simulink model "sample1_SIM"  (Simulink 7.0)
settings: Solver=ode3  StartTime=0.0  StopTime=70  RelTol=1e-3
libraries: simulink x6

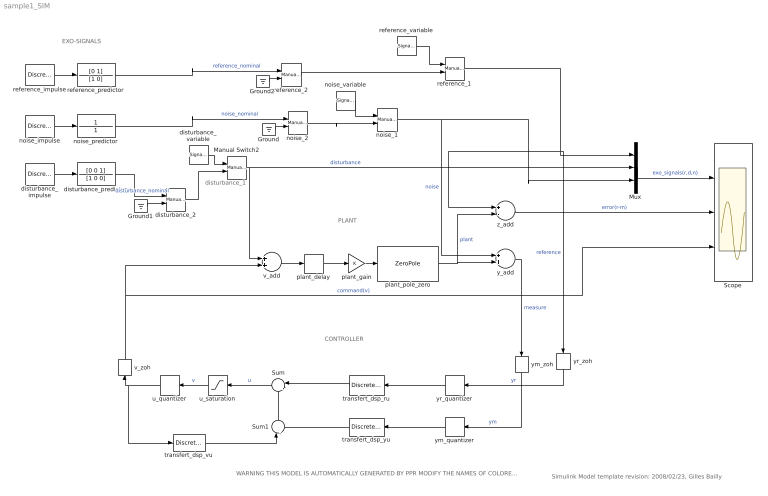
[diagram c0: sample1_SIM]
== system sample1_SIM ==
  note: PLANT
  note: EXO-SIGNALS
  note: Simulink Model template revision: 2008/02/23, Gilles Bailly
  note: CONTROLLER
  note: WARNING THIS MODEL IS AUTOMATICALLY GENERATED BY PPR MODIFY THE NAMES OF COLORED BLOCKS BREAK THIS LINK
  note: disturbance_1
  Ground : Ground
  Ground1 : Ground
  Ground2 : Ground
  Manual Switch2 : simulink/Signal Routing/Manual Switch  SystemSampleTime=-1  sw=0  action=0  varsize=off
  Mux : Mux  Inputs=3
  Scope : Scope  NumInputPorts=3
  Sum : Sum  Orientation=left  Inputs=|+-  OutDataType=sfix(16)  OutScaling=2^0
  Sum1 : Sum  Orientation=up  Inputs=|++  OutDataType=sfix(16)  OutScaling=2^0
  disturbance_2 : simulink/Signal Routing/Manual Switch  SystemSampleTime=-1  sw=1  action=0  varsize=off
  disturbance_impulse : DiscretePulseGenerator  Period=500  PhaseDelay=100  SampleTime=0.1
  disturbance_predictor : TransferFcn  Numerator=[0 0 1]  Denominator=[1 0 0]
  disturbance_variable : SignalGenerator
  noise_1 : simulink/Signal Routing/Manual Switch  SystemSampleTime=-1  sw=0  action=0  varsize=off
  noise_2 : simulink/Signal Routing/Manual Switch  SystemSampleTime=-1  sw=1  action=0  varsize=off
  noise_impulse : DiscretePulseGenerator  Period=500  PhaseDelay=200  SampleTime=0.1
  noise_predictor : TransferFcn  Numerator=1  Denominator=1
  noise_variable : SignalGenerator
  plant_delay : TransportDelay  DelayTime=0.5
  plant_gain : Gain  ParameterDataType=sfix(16)  ParameterScaling=2^0  OutDataType=sfix(16)  OutScaling=2^0
  plant_pole_zero : ZeroPole  Zeros=zeros(0,1)  Poles=-1  Gain=1
  reference_1 : simulink/Signal Routing/Manual Switch  SystemSampleTime=-1  sw=0  action=0  varsize=off
  reference_2 : simulink/Signal Routing/Manual Switch  SystemSampleTime=-1  sw=1  action=0  varsize=off
  reference_impulse : DiscretePulseGenerator  Period=500  PhaseDelay=10  SampleTime=0.1
  reference_predictor : TransferFcn  Numerator=[0 1]  Denominator=[1 0]
  reference_variable : SignalGenerator
  transfert_dsp_ru : DiscreteFilter  Orientation=left  Numerator=[0 0.7104960446]  Denominator=[1 -0.7408182207]  SampleTime=0.1
  transfert_dsp_vu : DiscreteFilter  Numerator=[0 0.1657069833 -0.2998382185 0.1356354391 7.122080703e-014 6.4420691e-014 5.825895322e-014 -0.07062683959 0.06825879814]  Denominator=[1 -2.714285714 2.455782313 -0.740632761 0 0 0 0 0]  SampleTime=0.1
  transfert_dsp_yu : DiscreteFilter  Orientation=left  Numerator=[0 0.7421702746 -1.388829544 0.6490273109]  Denominator=[1 -2.714285714 2.455782313 -0.740632761]  SampleTime=0.1
  u_quantizer : Quantizer  Orientation=left  QuantizationInterval=eps
  u_saturation : Saturate  Orientation=left  UpperLimit=10  LowerLimit=-10
  v_add : Sum  OutDataType=sfix(16)  OutScaling=2^-10
  v_zoh : ZeroOrderHold  Orientation=up  SampleTime=0.1
  y_add : Sum  OutDataType=sfix(16)  OutScaling=2^-10
  ym_quantizer : Quantizer  Orientation=left  QuantizationInterval=eps
  ym_zoh : ZeroOrderHold  Orientation=down  SampleTime=0.1
  yr_quantizer : Quantizer  Orientation=left  QuantizationInterval=eps
  yr_zoh : ZeroOrderHold  Orientation=down  SampleTime=0.1
  z_add : Sum  Inputs=+-  OutDataType=sfix(16)  OutScaling=2^-10
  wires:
  v_add/1 -> plant_delay/1
  y_add/1 -> ym_zoh/1  "measure"
  reference_impulse/1 -> reference_predictor/1
  noise_impulse/1 -> noise_predictor/1
  disturbance_impulse/1 -> disturbance_predictor/1
  plant_delay/1 -> plant_gain/1
  plant_gain/1 -> plant_pole_zero/1
  plant_pole_zero/1 -> y_add/2, z_add/2  "plant"
  transfert_dsp_vu/1 -> Sum1/1
  transfert_dsp_yu/1 -> Sum1/2
  Sum1/1 -> Sum/2
  yr_zoh/1 -> yr_quantizer/1  "yr"
  ym_zoh/1 -> ym_quantizer/1  "ym"
  Sum/1 -> u_saturation/1  "u"
  u_saturation/1 -> u_quantizer/1  "v"
  v_zoh/1 -> v_add/2, Scope/3  "command(v)"
  Mux/1 -> Scope/1  "exo_signals(r,d,n)"
  z_add/1 -> Scope/2  "error(r-m)"
  reference_1/1 -> Mux/1, yr_zoh/1, z_add/1  "reference"
  noise_1/1 -> Mux/3, y_add/1  "noise"
  Manual Switch2/1 -> v_add/1, Mux/2  "disturbance"
  reference_variable/1 -> reference_1/1
  noise_variable/1 -> noise_1/1
  disturbance_variable/1 -> Manual Switch2/1
  yr_quantizer/1 -> transfert_dsp_ru/1
  ym_quantizer/1 -> transfert_dsp_yu/1
  u_quantizer/1 -> v_zoh/1, transfert_dsp_vu/1
  transfert_dsp_ru/1 -> Sum/1
  noise_2/1 -> noise_1/2
  noise_predictor/1 -> noise_2/1  "noise_nominal"
  Ground/1 -> noise_2/2
  disturbance_predictor/1 -> disturbance_2/1  "disturbance_nominal"
  Ground1/1 -> disturbance_2/2
  disturbance_2/1 -> Manual Switch2/2
  reference_2/1 -> reference_1/2
  reference_predictor/1 -> reference_2/1  "reference_nominal"
  Ground2/1 -> reference_2/2
